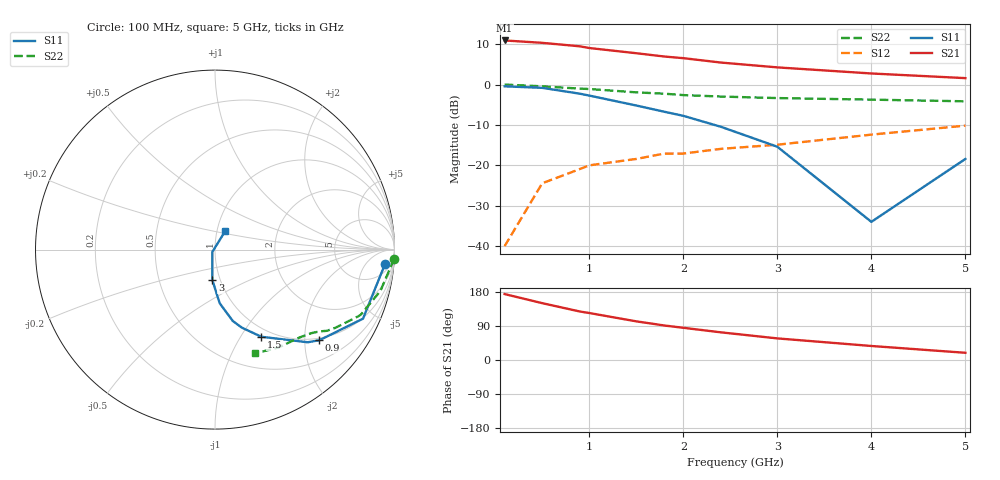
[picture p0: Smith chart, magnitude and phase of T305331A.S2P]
!AT-30533
!S and NOISE PARAMETERS at Vce=1V  Ic=1mA.  LAST UPDATED 06-23-94
# ghz s ma r 50!
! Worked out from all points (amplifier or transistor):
!   11 points, 100 MHz to 5 GHz, reference 50 ohm
!   highest |S21| = 10.9 dB at 100 MHz (marker M1)
!   |S21| within 3 dB of that: start of sweep to 1.439 GHz
!   unconditionally stable (mu >= 1): 2.505 GHz to 4.613 GHz
!   at 500 MHz: K = 0.26, MSG = 17.4 dB, |S12| = -24.4 dB
!   at 1.8 GHz: K = 0.80, MSG = 12.0 dB, |S12| = -17.1 dB
!   at 5 GHz: K = 0.98, MSG = 5.9 dB, |S12| = -10.2 dB
!   lowest NFmin = 0.30 dB at 500 MHz
!   S11 on the Smith chart (normalised r, x): 100 MHz: 10, -17; 900 MHz: 0.95, -2.35; 1.5 GHz: 0.89, -1.24; 3 GHz: 0.92, -0.32; 5 GHz: 1.10, +0.23
0.1  0.95 -5.0  3.51 174.0  0.01 87.0  0.999 -3.0
0.5  0.91 -25.0  3.28 150.0  0.06 73.0  0.95 -14.0
0.9  0.77 -41.0  2.97 128.0  0.09 63.0  0.89 -24.0
1  0.73 -45.0  2.83 124.0  0.1 61.0  0.88 -25.0
1.5  0.55 -62.0  2.44 102.0  0.12 54.0  0.8 -33.0
1.8  0.46 -71.0  2.22 91.0  0.14 51.0  0.77 -36.0
2  0.41 -76.0  2.12 85.0  0.14 50.0  0.74 -38.0
2.4  0.3 -85.0  1.87 73.0  0.16 49.0  0.71 -41.0
3  0.17 -95.0  1.63 57.0  0.18 49.0  0.68 -46.0
4  0.02 -139.0  1.37 37.0  0.24 48.0  0.65 -57.0
5  0.12 61.0  1.2 19.0  0.31 45.0  0.62 -69.0
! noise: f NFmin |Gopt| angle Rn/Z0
0.5  0.3  0.94  7  1.02
0.9  0.4  0.89  16  0.86
1.8  0.9  0.75  43  0.58
2.4  1.3  0.65  65  0.38
